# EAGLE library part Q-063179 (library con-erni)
Male Connector SMC-Q 12 contacts Standard Assembly Height Source: http://www.erni.com/DB/PDF-Drawing/SMC/063179.pdf
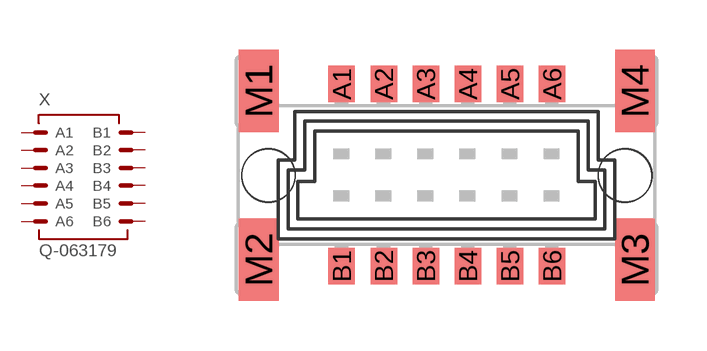
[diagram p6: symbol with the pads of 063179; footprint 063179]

Designator prefix X

## Q-063179 (OC_FARNELL: unknown; OC_NEWARK: unknown)  [063179]
A1  A1  pas
A2  A2  pas
A3  A3  pas
A4  A4  pas
A5  A5  pas
A6  A6  pas
B1  B1  pas
B2  B2  pas
B3  B3  pas
B4  B4  pas
B5  B5  pas
B6  B6  pas

## Footprint 063179 (pad centres in mm)
Male Connector SMC-Q 12 contacts Standard Assembly Height Source: http://www.erni.com/DB/PDF-Drawing/SMC/063179.pdf
smd 0.8 x 1.1: A1 -3.175,2.765; A2 -1.905,2.765; A3 -0.635,2.765; A4 0.635,2.765; A5 1.905,2.765; A6 3.175,2.765; B1 -3.175,-2.74; B2 -1.905,-2.74; B3 -0.635,-2.74; B4 0.635,-2.74; B5 1.905,-2.74; B6 3.175,-2.74
smd 1.2 x 2.5: M1 -5.68,2.55; M2 -5.68,-2.55; M3 5.68,-2.55; M4 5.68,2.55
hole 1.6 at -5.385,0
hole 1.6 at 5.385,0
